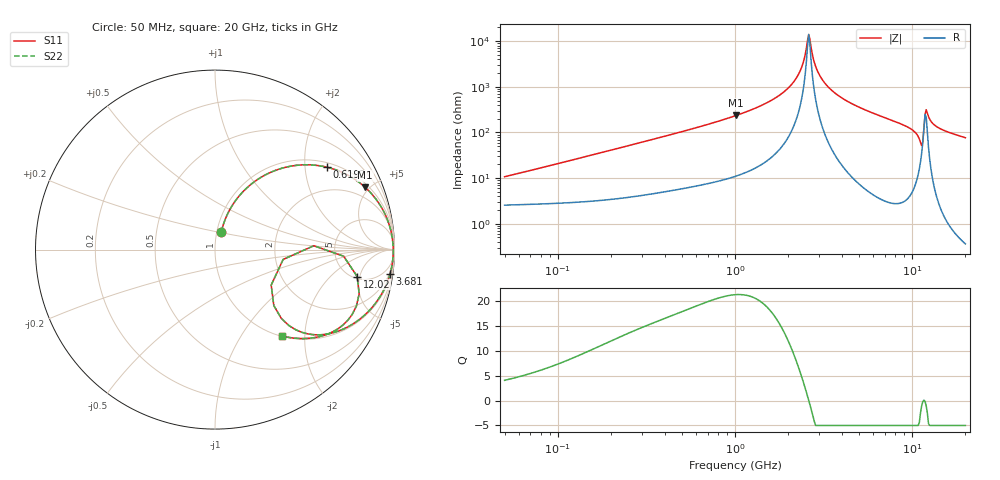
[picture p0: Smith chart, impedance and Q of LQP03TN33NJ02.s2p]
!Murata Part Number: LQP03TN33NJ02
!These Parameters are Measured in Series Mode Connection
!  o--[Z]--o
!Port1  Port2
!  o-------o
!Freq. Start=50[MHz] Stop=20[GHz], 401[Steps]
# Hz S RI R 50
!Freq.(Hz) S11(Real) S11(Imag) S21(Real) S21(Imag) S12(Real) S12(Imag) S22(Real) S22(Imag)
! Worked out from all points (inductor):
!   401 points, 50 MHz to 20 GHz, reference 50 ohm
!   read as one part in series: L = 32.9 nH near 51.52 MHz
!   highest Q = 21.3 at 1.015 GHz (marker M1), where L = 36.9 nH
!   self-resonance near 2.608 GHz
!   S11 on the Smith chart (normalised r, x): 50 MHz: 1.05, +0.21; 619.2 MHz: 1.14, +2.61; 3.681 GHz: 2, -14; 12.02 GHz: 5.32, -4.58; 20 GHz: 1.01, -1.53
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5e7  0.0348 0.0978  0.9652 -0.0978  0.9652 -0.0978  0.0348 0.0978
1.364002e8  0.096 0.2458  0.904 -0.2458  0.904 -0.2458  0.096 0.2458
3.721004e8  0.3772 0.4545  0.6228 -0.4545  0.6228 -0.4545  0.3772 0.4545
6.192061e8  0.6245 0.4588  0.3755 -0.4588  0.3755 -0.4588  0.6245 0.4588
1e9  0.8311 0.3519  0.1689 -0.3519  0.1689 -0.3519  0.8311 0.3519
1.015091e9  0.8364 0.3472  0.1636 -0.3472  0.1636 -0.3472  0.8364 0.3472
1.875929e9  0.9742 0.1269  0.0258 -0.1269  0.0258 -0.1269  0.9742 0.1269
2.279204e9  0.9894 0.0523  0.0106 -0.0523  0.0106 -0.0523  0.9894 0.0523
2.419936e9  0.9917 0.0292  0.00831 -0.0292  0.00831 -0.0292  0.9917 0.0292
2.569357e9  0.9928 0.0061  0.00717 -0.0061  0.00717 -0.0061  0.9928 0.0061
2.647493e9  0.993 -0.00548  0.00702 0.00548  0.00702 0.00548  0.993 -0.00548
2.728004e9  0.9928 -0.0171  0.00715 0.0171  0.00715 0.0171  0.9928 -0.0171
3.029571e9  0.9902 -0.0578  0.00983 0.0578  0.00983 0.0578  0.9902 -0.0578
3.680849e9  0.9756 -0.1341  0.0244 0.1341  0.0244 0.1341  0.9756 -0.1341
7.442007e9  0.7857 -0.403  0.2143 0.403  0.2143 0.403  0.7857 -0.403
1.019291e10  0.5385 -0.473  0.4615 0.473  0.4615 0.473  0.5385 -0.473
1.115139e10  0.3277 -0.312  0.6723 0.312  0.6723 0.312  0.3277 -0.312
1.166392e10  0.5504 0.0214  0.4496 -0.0214  0.4496 -0.0214  0.5504 0.0214
1.201863e10  0.7925 -0.1504  0.2075 0.1504  0.2075 0.1504  0.7925 -0.1504
1.257102e10  0.7639 -0.3621  0.2361 0.3621  0.2361 0.3621  0.7639 -0.3621
1.354865e10  0.6563 -0.4578  0.3437 0.4578  0.3437 0.4578  0.6563 -0.4578
2e10  0.3712 -0.4808  0.6288 0.4808  0.6288 0.4808  0.3712 -0.4808
